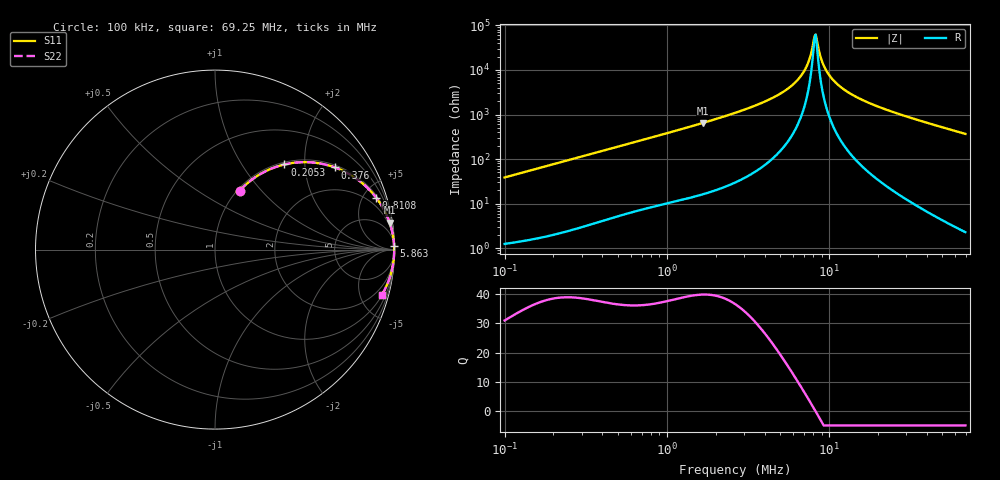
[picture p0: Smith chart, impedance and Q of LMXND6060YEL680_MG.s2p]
! LMXND6060YEL680_MG  S-PARAMETER MODEL  ( General Type )
! Model Generated by TAIYO YUDEN Corporation (http://www.ty-top.com)
! Version 1.0
! TAIYO YUDEN Control No. 191025NI43SB-FBB
! Copyright(c) 2019 TAIYO YUDEN CO.,LTD. All Rights Reserved.
! Product Description (link to TY-COMPAS)
! https://ds.yuden.co.jp/TYCOMPAS/or/detail?pn=LMXND6060YEL680MMG&u=M
! Products Name : Inductors
! Characteristics :
!  Inductance : 68 uH , SRF(min) : 4.0 MHz , DC Resistance(max) : 0.3952 Ohm
!  Rated Current : Saturation :1100 mA , Temp Rise : 950 mA
!  Case Size : 6.0 x 6.0 / 0.236 x 0.236 [mm/inch] , Thickness : 4.5 / 0.177 [mm/inch]
!  (Conditions: Temperature = 25 degC , DC Bias Current/Voltage = 0A / 0V)
! External Node Assignments :
!  1  o---GGG---o  2
! GND o---------o GND
! Frequency Range : 0.1MHz  -  69.245953MHz  [ 402 STEP ]
# MHz S RI R 50
! Freq[MHz].  S11 Real  S11 Imag  S21 Real  S21 Imag  S12 Real  S12 Imag  S22 Real  S22 Imag
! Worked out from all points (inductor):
!   401 points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, 100 kHz to 69.25 MHz, reference 50 ohm
!   read as one part in series: L = 61.4 uH near 103.3 kHz
!   highest Q = 39.9 at 1.665 MHz (marker M1), where L = 61.7 uH
!   self-resonance near 8.131 MHz
!   S11 on the Smith chart (normalised r, x): 100 kHz: 1.02, +0.77; 205.3 kHz: 1.04, +1.58; 376 kHz: 1.08, +2.87; 810.8 kHz: 1.17, +6.15; 5.863 MHz: 8, +88; 69.25 MHz: 1.05, -7.34
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0.1  0.1381 0.3292  0.8619 -0.3292  0.8619 -0.3292  0.1381 0.3292
0.205326  0.3863 0.4741  0.6137 -0.4741  0.6137 -0.4741  0.3863 0.4741
0.299065  0.5655 0.4829  0.4345 -0.4829  0.4345 -0.4829  0.5655 0.4829
0.375993  0.6691 0.4575  0.3309 -0.4575  0.3309 -0.4575  0.6691 0.4575
0.810823  0.898 0.2893  0.102 -0.2893  0.102 -0.2893  0.898 0.2893
0.894401  0.914 0.2672  0.086 -0.2672  0.086 -0.2672  0.914 0.2672
1.664829  0.973 0.1502  0.027 -0.1502  0.027 -0.1502  0.973 0.1502
2.631463  0.9892 0.0908  0.0108 -0.0908  0.0108 -0.0908  0.9892 0.0908
4.297608  0.9961 0.0455  0.00394 -0.0455  0.00394 -0.0455  0.9961 0.0455
5.863346  0.9978 0.0226  0.0022 -0.0226  0.0022 -0.0226  0.9978 0.0226
7.134398  0.9983 0.0094  0.0017 -0.0094  0.0017 -0.0094  0.9983 0.0094
7.493079  0.9984 0.00616  0.00164 -0.00616  0.00164 -0.00616  0.9984 0.00616
7.869792  0.9984 0.00295  0.0016 -0.00295  0.0016 -0.00295  0.9984 0.00295
8.131398  0.9984 0.000804  0.00158 -0.000804  0.00158 -0.000804  0.9984 0.000804
8.265445  0.9984 -0.000266  0.00158 0.000266  0.00158 0.000266  0.9984 -0.000266
8.401701  0.9984 -0.00134  0.00157 0.00134  0.00157 0.00134  0.9984 -0.00134
8.96956  0.9984 -0.00562  0.00159 0.00562  0.00159 0.00562  0.9984 -0.00562
9.575801  0.9984 -0.00994  0.00165 0.00994  0.00165 0.00994  0.9984 -0.00994
11.65164  0.9979 -0.0232  0.00206 0.0232  0.00206 0.0232  0.9979 -0.0232
15.38522  0.9966 -0.0436  0.00341 0.0436  0.00341 0.0436  0.9966 -0.0436
23.53582  0.9918 -0.0816  0.00822 0.0816  0.00822 0.0816  0.9918 -0.0816
69.24595  0.9296 -0.2528  0.0704 0.2528  0.0704 0.2528  0.9296 -0.2528
